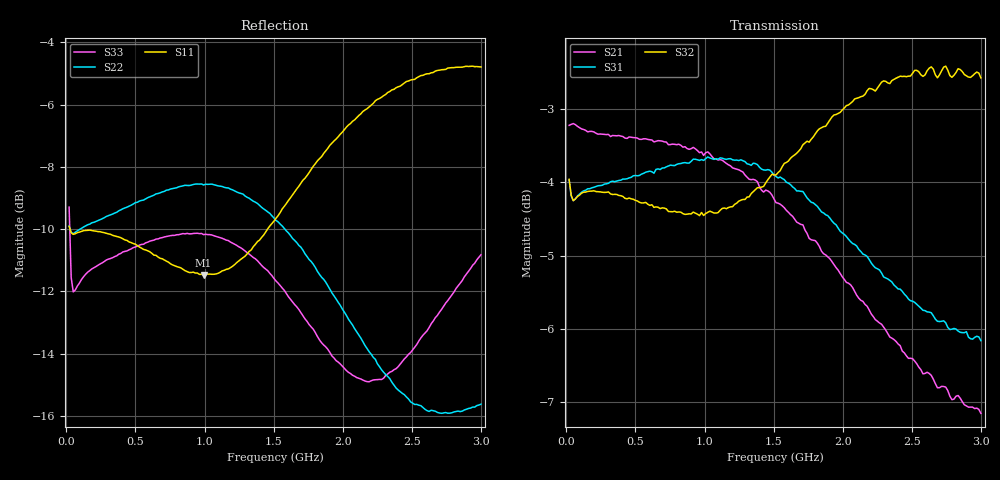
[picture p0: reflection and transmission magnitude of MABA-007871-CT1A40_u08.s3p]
#	MHz	S	RI	R	50
!FREQ	R1	I1	R2	I2	R3	I3
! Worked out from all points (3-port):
!   200 points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, 19.98 MHz to 3 GHz, reference 50 ohm
!   strongest paths, dB at 19.98 MHz, 768.7 MHz, 1.517 GHz, 2.266 GHz, 3 GHz:
!     S32: -4.0, -4.4, -3.9, -2.7, -2.6
!     S31: -4.0, -3.8, -3.9, -5.2, -6.2
!     S21: -3.2, -3.5, -4.3, -5.9, -7.1
!   lowest |S11| = -11.5 dB at 993.4 MHz (marker M1), VSWR 1.73, Z = 36.4 - j19.4 ohm
!   |S11| at or under -10 dB: 26.61 MHz to 1.456 GHz (1.429 GHz wide, 193 % of centre)
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19.975  0.316 0.048  0.6861 -0.0731  -0.6254 -0.0992
        0.6862 -0.0729  0.3146 0.0584  0.6241 0.1107
        -0.6254 -0.0992  0.6244 0.1098  0.2538 0.2308
49.925  0.3101 -0.00209  0.6894 -0.0615  -0.613 -0.00739
        0.6892 -0.0612  0.31 0.0232  0.6121 0.0326
        -0.613 -0.00739  0.6122 0.0328  0.2334 0.0914
124.8  0.3105 -0.0498  0.6768 -0.1089  -0.6193 0.0637
       0.6769 -0.1086  0.3185 0.0137  0.6209 0.000305
       -0.6193 0.0637  0.6213 0.000793  0.2589 0.058
604  0.1451 -0.252  0.5232 -0.4312  -0.4982 0.4052
     0.5227 -0.4265  0.3548 -0.0325  0.6031 -0.0928
     -0.4982 0.4052  0.6014 -0.0927  0.3024 0.00662
993.35  -0.1016 -0.2467  0.2638 -0.6071  -0.2667 0.5962
        0.2701 -0.6003  0.3557 -0.11  0.5876 -0.1292
        -0.2667 0.5962  0.5849 -0.1293  0.3069 -0.0421
1517.475  -0.3227 0.065  -0.1678 -0.5804  0.1335 0.6226
          -0.1556 -0.591  0.2606 -0.1967  0.6154 -0.1884
          0.1335 0.6226  0.6096 -0.1893  0.2444 -0.0915
1831.95  -0.2642 0.314  -0.3577 -0.423  0.3232 0.5113
         -0.3586 -0.4436  0.1859 -0.1923  0.6388 -0.2661
         0.3232 0.5113  0.6342 -0.2624  0.1969 -0.0727
2251.25  0.00626 0.511  -0.4594 -0.1584  0.4522 0.3147
         -0.4785 -0.1687  0.1302 -0.1412  0.6218 -0.4034
         0.4522 0.3147  0.6161 -0.3945  0.1808 -0.0115
2610.65  0.2771 0.4887  -0.4452 0.0465  0.4887 0.162
         -0.4649 0.057  0.1272 -0.0996  0.5551 -0.5232
         0.4887 0.162  0.5538 -0.5084  0.2144 0.0337
3000  0.4868 0.3083  -0.3589 0.2355  0.492 0.0123
      -0.3584 0.2537  0.1436 -0.0822  0.4258 -0.6255
      0.492 0.0123  0.4255 -0.6096  0.2838 0.0465
